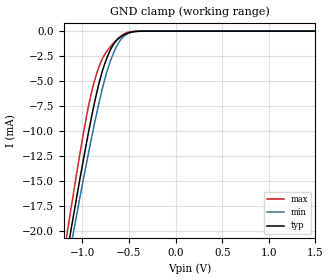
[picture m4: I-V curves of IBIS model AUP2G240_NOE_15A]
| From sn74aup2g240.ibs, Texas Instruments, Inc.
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[Model]   AUP2G240_NOE_15A
Model_type  Input
Vinl=0.56
Vinh=0.91
| variable   typ   min   max
C_comp   1.47pF   1.28pF   1.79pF
[Temperature Range]   40   100   -40
| Ambient temperature   25   85   -40
[Voltage range]   1.5   1.4   1.6
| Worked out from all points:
|   GND clamp passes 1 mA (typ) near -0.64 V on its own axis
[GND Clamp]
| AUP2G240_NOE_15A
|   Voltage   I(typ)   I(min)   I(max)
-3.6V     -169.6mA   -161.4mA   -179.1mA
-1.16V    -21.94mA   -23.37mA   -19.97mA
-1.11V    -19.21mA   -20.81mA   -17.01mA
-1.09V    -18.13mA   -19.79mA   -15.84mA
-955mV    -11.11mA   -13.14mA   -8.466mA
-850mV    -6.292mA   -8.346mA   -4.331mA
-785mV    -3.967mA   -5.715mA   -2.747mA
-710mV    -2.081mA   -3.263mA   -1.67mA
-635mV    -950.3uA   -1.567mA   -878.7uA
-550mV    -358.9uA   -461.1uA   -270.7uA
-330mV    -2.909uA   -4.627uA   -452.5nA
1.5V      74.87pA    433.8pA    15.81pA
